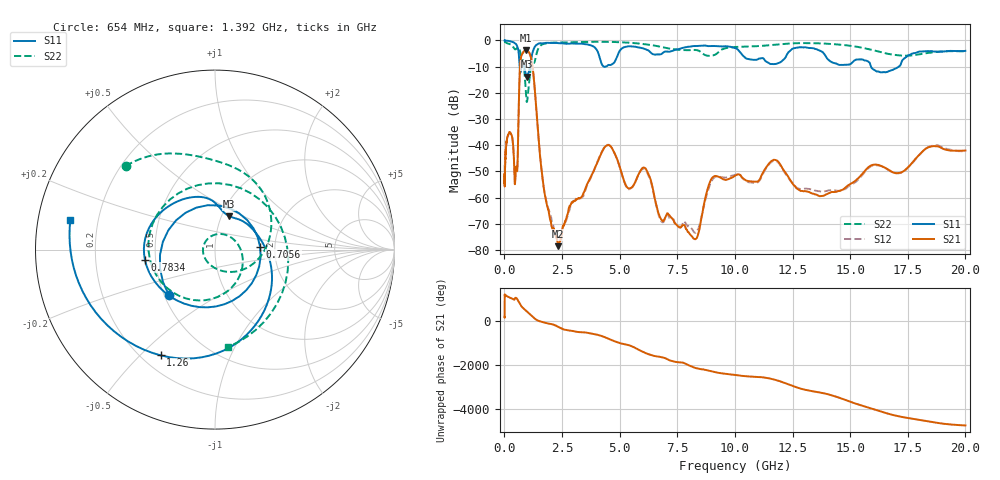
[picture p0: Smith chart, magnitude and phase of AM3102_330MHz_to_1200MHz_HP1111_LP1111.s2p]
! Date/Time: Tue, Sep 11, 2018 5:24 PM
! Network Analyzer: Agilent Technologies E8362B Rev: A.07.50.63
! Sweep from 0.010 to 20.000 GHz, 1601 Points, Sweep Type: LOG
! Power Supply: 4.949 V, 0.001 A
# Hz S DB R 50
!freq MagS11 AngS11 MagS21 AngS21 MagS12 AngS12 MagS22 AngS22
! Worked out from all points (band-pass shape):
!   1601 points, 10 MHz to 20 GHz, reference 50 ohm
!   highest |S21| = -3.62 dB at 933.9 MHz (marker M1); lowest = -78.5 dB at 2.336 GHz (marker M2)
!   |S21| within 3 dB of the highest: 715.5 MHz to 1.155 GHz (439.3 MHz wide, 47 % of centre)
!   lowest |S11| = -13.9 dB at 960.9 MHz (marker M3), VSWR 1.51, Z = 54.4 + j21.1 ohm
!   |S11| at or under -10 dB: 661.7 MHz to 736.2 MHz (74.46 MHz wide, 10.7 % of centre); 858.7 MHz to 1.108 GHz (248.9 MHz wide, 25.3 % of centre); 15.91 GHz to 17.11 GHz (1.206 GHz wide, 7.3 % of centre)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
!   |S22| runs from -23.5 to -0.2 dB; largest |S21 - S12| = 0.008
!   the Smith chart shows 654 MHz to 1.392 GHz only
!   S11 on the Smith chart (normalised r, x): 654 MHz: 0.53, -0.31; 705.6 MHz: 1.67, +0.05; 783.4 MHz: 0.44, -0.06; 1.26 GHz: 0.27, -0.58; 1.392 GHz: 0.10, +0.10
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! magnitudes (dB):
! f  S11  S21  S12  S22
! 10 MHz  0.0  -50.9  -47.5  -0.2
! 35.55 MHz  -0.1  -47.1  -46.8  -0.5
! 126.4 MHz  -0.2  -37.2  -37.2  -1.1
! 334.7 MHz  -0.6  -36.8  -36.8  -1.9
! 447.2 MHz  -1.0  -54.2  -53.9  -3.3
! 564.4 MHz  -2.4  -48.7  -48.5  -2.8
! 654 MHz  -8.9  -15.0  -15.1  -3.3
! 705.6 MHz  -12.0  -7.2  -7.2  -5.3
! 783.4 MHz  -8.1  -5.0  -5.0  -7.1
! 933.9 MHz  -13.3  -3.6  -3.7  -20.6
! 960.9 MHz  -13.9  -3.7  -3.8  -23.2
! 1.26 GHz  -3.6  -12.9  -12.9  -8.6
! 1.392 GHz  -1.7  -26.9  -27.4  -5.2
! 1.59 GHz  -1.1  -47.7  -47.7  -1.8
! 2.336 GHz  -1.0  -78.5  -75.5  -0.8
! 4.415 GHz  -9.9  -40.2  -40.1  -0.5
! 5.652 GHz  -2.4  -54.5  -54.6  -1.0
! 8.149 GHz  -2.2  -75.0  -72.1  -3.7
! 9.22 GHz  -2.2  -51.8  -52.0  -5.0
! 11.75 GHz  -9.0  -45.6  -45.8  -1.6
! 13.94 GHz  -6.0  -58.8  -57.5  -1.2
! 20 GHz  -4.0  -42.0  -42.5  -4.1
